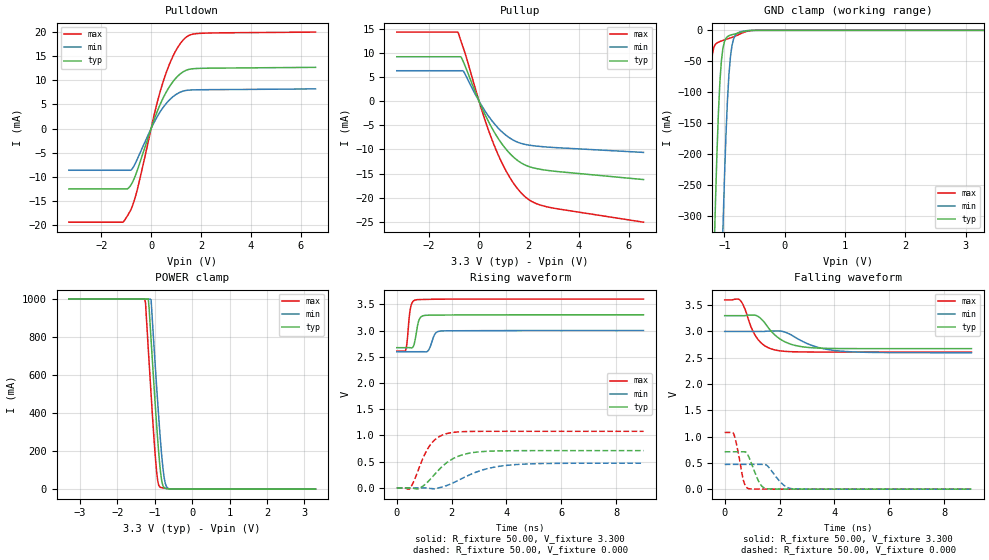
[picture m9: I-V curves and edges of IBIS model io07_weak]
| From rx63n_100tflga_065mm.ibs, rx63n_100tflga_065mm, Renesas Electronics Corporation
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[Model]   io07_weak
Model_type   I/O
Polarity   Non-Inverting
Enable   Active-High
Vinl  =   0.660V
Vinh  =   2.640V
Vmeas =   1.650V
Cref  =   30.00pF
| variable   typ   min   max
C_comp   3.960pF   3.960pF   3.960pF
| variable   typ   min   max
[Temperature Range]   45.000   105.000   -40.000
| variable   typ   min   max
[Voltage Range]   3.300V   3.000V   3.600V
| variable   typ   min   max
[Pullup Reference]   3.300V   3.000V   3.600V
| variable   typ   min   max
[Pulldown Reference]   0.000V   0.000V   0.000V
| variable   typ   min   max
[POWER Clamp Reference] 3.300V   3.000V   3.600V
| variable   typ   min   max
[GND Clamp Reference]   0.000V   0.000V   0.000V
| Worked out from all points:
|   slope of the pulldown table from 0 to 0.495 V, typ, clamps not added: 76.6 ohm
|   slope of the pullup table from 0 to 0.495 V, typ, clamps not added: 92.4 ohm
|   GND clamp passes 1 mA (typ) near -0.63 V on its own axis
|   POWER clamp passes 1 mA (typ) near -0.58 V on its own axis
|   rising waveform, R_fixture 50.00, V_fixture 3.300: 20-80 % time 135ps typ, 167ps min, 111ps max; typ from 2.67 V to 3.3 V
|   rising waveform, R_fixture 50.00, V_fixture 0.000: 20-80 % time 910ps typ, 1.34ns min, 595ps max; typ from 0 V to 0.711 V
|   falling waveform, R_fixture 50.00, V_fixture 3.300: 20-80 % time 770ps typ, 1.08ns min, 526ps max; typ from 3.3 V to 2.67 V
|   falling waveform, R_fixture 50.00, V_fixture 0.000: 20-80 % time 331ps typ, 446ps min, 234ps max; typ from 0.711 V to 0 V
[Pulldown]
| io07_weak Pulldown rx631_rx63n
| Thu Mar 22 17:15:49 2012
| voltage   I(typ)   I(min)   I(max)
-3.3V     -12.52mA   -8.65mA    -19.42mA
-1.15V    -12.52mA   -8.65mA    -19.42mA
-1.025V   -12.52mA   -8.65mA    -18.72mA
-800mV    -11.64mA   -8.594mA   -16.68mA
-600mV    -9.336mA   -6.851mA   -13.58mA
175mV     2.596mA    1.815mA    3.964mA
525mV     6.766mA    4.671mA    10.37mA
950mV     10.19mA    6.891mA    15.75mA
1.4V      12.07mA    7.901mA    18.93mA
1.7V      12.42mA    8.02mA     19.61mA
2.1V      12.5mA     8.057mA    19.78mA
6.6V      12.7mA     8.228mA    20.01mA
[Pullup]
| io07_weak Pullup rx631_rx63n
| Thu Mar 22 17:15:49 2012
| voltage   I(typ)   I(min)   I(max)
-3.3V     9.166mA    6.276mA    14.26mA
-850mV    9.166mA    6.276mA    14.26mA
-725mV    9.114mA    6.276mA    12.4mA
-625mV    8.067mA    6.148mA    10.91mA
175mV     -2.054mA   -1.515mA   -2.91mA
700mV     -7.168mA   -5.188mA   -10.28mA
1.025V    -9.573mA   -6.827mA   -13.86mA
1.325V    -11.3mA    -7.926mA   -16.53mA
1.95V     -13.44mA   -9.058mA   -20.2mA
2.3V      -13.95mA   -9.303mA   -21.2mA
2.9V      -14.43mA   -9.565mA   -22.05mA
6.6V      -16.23mA   -10.61mA   -25.04mA
[GND Clamp]
| io07_weak GNDClamp rx631_rx63n
| Thu Mar 22 17:15:49 2012
| voltage   I(typ)   I(min)   I(max)
-3.3V     -1A        -1A        -1A
-1.325V   -1A        -1A        -369.2mA
-1.3V     -928.6mA   -1A        -269.7mA
-1.25V    -694.8mA   -1A        -112.6mA
-1.175V   -376mA     -953.3mA   -27.44mA
-1.15V    -283.8mA   -837.7mA   -22.69mA
-1.075V   -83.42mA   -512.2mA   -18.16mA
-1.025V   -28.94mA   -323mA     -16.39mA
-925mV    -8.707mA   -71.38mA   -13.1mA
-850mV    -6.468mA   -14.65mA   -10.64mA
-675mV    -1.81mA    -1.082mA   -3.186mA
3.3V      0A         0A         0A
[POWER Clamp]
| io07_weak PWRClamp rx631_rx63n
| Thu Mar 22 17:15:49 2012
| voltage   I(typ)   I(min)   I(max)
-3.3V     1A         1A         1A
-1.275V   1A         1A         1A
-1.25V    1A         1A         982.1mA
-1.175V   1A         1A         736.6mA
-1.1V     784.3mA    995.9mA    498mA
-1V       476.2mA    683.1mA    204.7mA
-950mV    332.1mA    533mA      87.52mA
-875mV    143.3mA    321.7mA    12.76mA
-825mV    55.42mA    197.2mA    7.873mA
-750mV    8.12mA     59.94mA    5.513mA
-625mV    1.619mA    2.607mA    2.132mA
3.3V      0A         0A         0A
[Ramp]
dV/dt_r   0.427/910.44p  0.283/1.34n   0.648/594.54p
dV/dt_f   0.376/770.72p  0.242/1.09n   0.595/525.58p
R_load = 50.00ohm
[Rising Waveform]
| io07_weak Rising-High rx631_rx63n
| Thu Mar 22 17:15:49 2012
R_fixture = 50.00
V_fixture = 3.300
V_fixture_min = 3.000
V_fixture_max = 3.600
C_fixture = 0.00pF
| Time   V(typ)   V(min)   V(max)
0s        2.673V     2.596V     2.608V
325ps     2.673V     2.596V     2.63V
495ps     2.672V     2.596V     3.414V
605ps     2.7V       2.596V     3.562V
690ps     2.883V     2.596V     3.584V
825ps     3.217V     2.596V     3.59V
1.05ns    3.29V      2.593V     3.593V
1.4ns     3.294V     2.941V     3.597V
1.65ns    3.295V     2.993V     3.598V
9ns       3.3V       3V         3.6V
[Rising Waveform]
| io07_weak Rising-Low rx631_rx63n
| Thu Mar 22 17:15:49 2012
R_fixture = 50.00
V_fixture = 0.000
C_fixture = 0.00pF
| Time   V(typ)   V(min)   V(max)
0s        0V         0V         0V
465ps     1mV        0V         -19mV
790ps     -19mV      0V         347mV
1ns       53mV       0V         619mV
1.18ns    141mV      -7mV       789mV
1.475ns   312mV      -6mV       953mV
1.85ns    492mV      51mV       1.039V
2.605ns   658mV      237mV      1.076V
3.935ns   707mV      425mV      1.079V
9ns       711mV      471mV      1.079V
[Falling Waveform]
| io07_weak Falling-High rx631_rx63n
| Thu Mar 22 17:15:49 2012
R_fixture = 50.00
V_fixture = 3.300
V_fixture_min = 3.000
V_fixture_max = 3.600
C_fixture = 0.00pF
| Time   V(typ)   V(min)   V(max)
0s        3.3V       3V         3.6V
555ps     3.3V       3V         3.598V
695ps     3.299V     3V         3.481V
1.165ns   3.3V       3V         2.883V
1.46ns    3.164V     3.001V     2.728V
1.88ns    2.911V     3.009V     2.643V
2.65ns    2.725V     2.864V     2.612V
3.315ns   2.686V     2.711V     2.608V
4.13ns    2.675V     2.631V     2.608V
9ns       2.673V     2.596V     2.608V
[Falling Waveform]
| io07_weak Falling-Low rx631_rx63n
| Thu Mar 22 17:15:49 2012
R_fixture = 50.00
V_fixture = 0.000
C_fixture = 0.00pF
| Time   V(typ)   V(min)   V(max)
0s        711mV      471mV      1.079V
335ps     711mV      471mV      1.044V
450ps     711mV      471mV      807mV
690ps     711mV      471mV      156mV
885ps     606mV      471mV      9mV
1.26ns    128mV      471mV      2mV
1.54ns    8mV        452mV      1mV
2.085ns   2mV        108mV      0V
2.46ns    1mV        8mV        0V
9ns       0V         0V         0V
